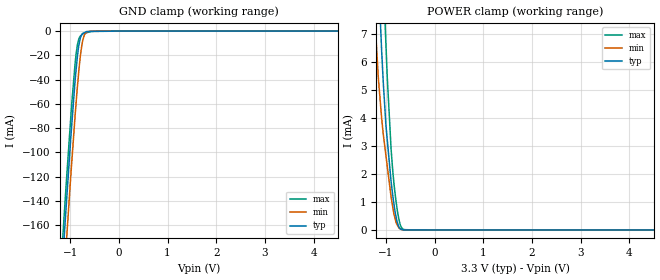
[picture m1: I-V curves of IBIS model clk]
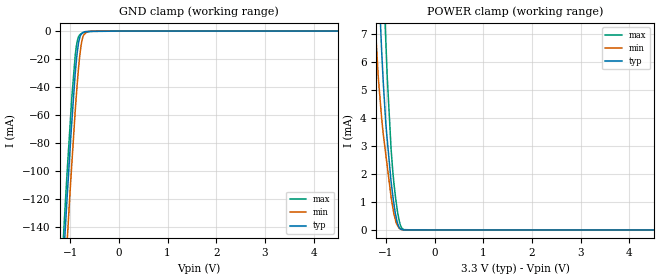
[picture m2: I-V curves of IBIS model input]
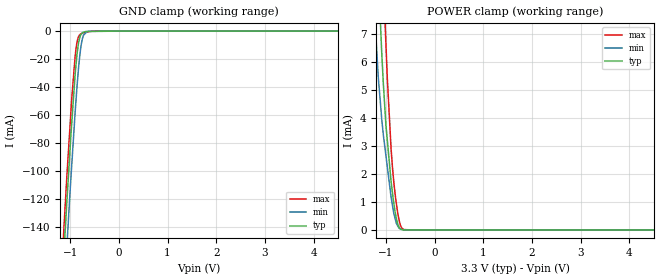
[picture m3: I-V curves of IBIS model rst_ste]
|Texas Instruments Incorporated
| A LOW COST INTEGRATED ANALOG FRONT END FOR WEIGH SCALE AND BODY COMPOSITION
| MEASUREMENT
| Marketing part#   Digital Voltage Range   Package-type   #pins
| AFE4300   2.0V - 3.6V   TQFP   80
[IBIS Ver]   3.2
[File name]   afe4300pn.ibs
[File Rev]   1.0
[Date]   6/8/2012
[Source]
| Texas Instruments Incorporated.
| Analog-eLab Design Center, HPA
| 12500 TI Blvd
| Dallas, TX -75243
| e-mail: elab_scm_ibis@list.ti.com
[Notes]   Revision History:
| Rev 1.0: 6/8/2012
| - Initial version of the model
| - Model generated from simulations in TISPICE
| - Model matched to SPICE simulation
| - C_comp although listed in numerical order of value are
|   obtained from varying PVT conditions. For PVT conditions for
|   each specific value refer the buffer description under
|   respective [Model]. IBIS model user is responsible for using
|   appropriate C_comp to simulate for Signal Integrity.
| - Model names with a trailing _3p3 contains the model for
|   3.3V [3.0V and 3.6V].
[Disclaimer]
| This model is designed as an aid for customers of Texas Instruments.
| TI and its licensors and suppliers make no warranties, either expressed
| or implied, with respect to this  model, including the warranties of
| merchantability or fitness for a particular purpose. The model is
| provided solely on an "as is" basis. The entire risk as to its quality
| and performance is with the customer.
[Copyright]
 (C) Copyright 2011 Texas Instruments Incorporated.All rights reserved.
|   AFE4300PN
[Component]   AFE4300PN
[Manufacturer]   TI
[Package]   |80 TQFP   -  PN package
|   typ   min   max
R_pkg   0.10791   0.08655   0.13328
L_pkg   4.92072nH   4.19191nH   6.00445nH
C_pkg   0.77225pF   0.63735pF   1.07420pF
[Pin]  signal_name   model_name   R_pin   L_pin   C_pin
1   AVSS   gnd   0.06488   4.97502nH  0.79351pF
2   INP1   term   0.12382   5.42900nH  0.85172pF
3   INM1   term   0.12069   5.27719nH  0.83213pF
4   INP2   term   0.11830   5.14232nH  0.81045pF
5   INM2   term   0.11658   5.03610nH  0.79047pF
6   AVSS   gnd   0.11574   4.97329nH  0.71405pF
7   INP_R   term   0.11479   4.85156nH  0.70853pF
8   INM_R   term   0.11470   4.77192nH  0.75908pF
9   AVSS   gnd   0.11737   5.96548nH  1.07056pF
10   INP3   term   0.11594   4.78579nH  0.68513pF
11   INM3   term   0.11660   4.80030nH  0.68657pF
12   INP4   term   0.11918   6.00445nH  1.07420pF
13   INM4   term   0.11809   4.84466nH  0.76427pF
14   AVSS   gnd   0.11963   4.95544nH  0.71226pF
15   AAUX   term   0.12075   5.08150nH  0.70418pF
16   VLDO   term   0.11317   4.96716nH  0.77207pF
17   VREF   term   0.11366   5.04855nH  0.80047pF
18   AVDD   power   0.11453   5.15212nH  0.81475pF
19   DACOUT   term   0.12377   5.43268nH  0.84789pF
20   DAC_FILT_IN   term   0.13328   5.76711nH  0.74859pF
21   AVSS   gnd   0.13115   5.73004nH  0.74408pF
22   IOUT5   term   0.12643   5.49576nH  0.86054pF
23   IOUT4   term   0.12223   5.32047nH  0.84033pF
24   IOUT3   term   0.11875   5.16170nH  0.81605pF
25   IOUT2   term   0.11590   5.03136nH  0.79392pF
26   IOUT1   term   0.11367   4.93832nH  0.71474pF
27   IOUT0   term   0.11178   4.79271nH  0.70623pF
28   RP1   term   0.11064   4.69143nH  0.75471pF
29   RP0   term   0.11208   5.85943nH  1.06436pF
30   RN1   term   0.10991   4.66416nH  0.67662pF
31   RN0   term   0.10965   4.65917nH  0.66509pF
32   AVSS   gnd   0.11258   5.87032nH  1.05278pF
33   VSENSE5   term   0.10888   4.65569nH  0.75096pF
34   VSENSE4   term   0.10764   4.70739nH  0.69961pF
35   VSENSE3   term   0.10712   4.79958nH  0.70339pF
36   VSENSE2   term   0.10696   4.84185nH  0.77759pF
37   VSENSE1   term   0.10745   4.92272nH  0.79503pF
38   VSENSE0   term   0.10865   5.03281nH  0.81479pF
39   VSENSEP_R1   term   0.11067   5.16161nH  0.83129pF
40   VSENSEP_R0   term   0.11360   5.35645nH  0.71822pF
41   VSENSEM_R1   term   0.10765   5.23060nH  0.71458pF
42   VSENSEM_R0   term   0.09674   4.87022nH  0.80715pF
43   NC   nc   0.09741   4.79802nH  0.79221pF
44   NC   nc   0.09371   4.63612nH  0.77888pF
45   AVSS   gnd   0.09092   4.50774nH  0.75677pF
46   AVDD   power   0.08905   4.42347nH  0.67917pF
47   OUTM_I_FILT   term   0.08798   4.29859nH  0.67325pF
48   OUTP_I_FILT   term   0.08732   4.20648nH  0.72239pF
49   OUTM_Q_FILT   term   0.08936   5.38610nH  1.03329pF
50   OUTP_Q_FILT   term   0.08789   4.20454nH  0.64654pF
51   AAUX2   term   0.08803   4.20667nH  0.63735pF
52   NC   nc   0.00742   3.98391nH  0.92611pF
53   _RESET   rst_ste   0.08675   4.19191nH  0.70875pF
54   STE   rst_ste   0.08674   4.26853nH  0.65925pF
55   NC   nc   0.00583   2.99607nH  0.56984pF
56   SDOUT   output   0.08722   4.42874nH  0.74037pF
57   SDIN   input   0.08862   4.52766nH  0.76099pF
58   SCLK   input   0.08655   4.57061nH  0.77680pF
59   RDY   output   0.08826   4.69216nH  0.79488pF
60   AVSS   gnd   0.08879   4.83658nH  0.67875pF
61   NC   nc   0.00646   3.43131nH  0.58837pF
62   NC   nc   0.00634   3.29482nH  0.69454pF
63   NC   nc   0.00622   3.20561nH  0.68015pF
64   NC   nc   0.00608   3.11757nH  0.66177pF
65   NC   nc   0.00595   3.04425nH  0.64463pF
66   NC   nc   0.00583   2.99602nH  0.56986pF
67   NC   nc   0.00536   2.86106nH  0.56090pF
68   NC   nc   0.00532   2.79061nH  0.60735pF
69   NC   nc   0.00733   3.97085nH  0.91820pF
70   NC   nc   0.00533   2.78774nH  0.53745pF
71   NC   nc   0.00536   2.79295nH  0.53912pF
72   NC   nc   0.08978   5.38902nH  1.01684pF
73   NC   nc   0.08745   4.20291nH  0.71651pF
74   NC   nc   0.08899   4.31242nH  0.66607pF
75   NC   nc   0.08705   4.37168nH  0.66100pF
76   NC   nc   0.00591   3.03491nH  0.64624pF
77   AVSS   gnd   0.08838   4.50833nH  0.74945pF
78   NC   nc   0.00613   3.18898nH  0.67809pF
79   CLK   clk   0.09735   4.85821nH  0.80082pF
80   AVDD   power   0.10961   5.24317nH  0.71225pF
[Model] term
Model_type Terminator
C_comp   1.0e-20F  1.0e-20F  1.0e-20F
|   typ   min   max
[Voltage Range]   3.3V   3.0V   3.6V
[POWER Clamp Reference]   3.3V   3.0V   3.6V
[GND Clamp Reference]   0V   0V   0V
|Ambient Temperature   25   70   0
|Junction Temperature
[Temperature Range]   27   70   0
| Models and submodels in the file (5): clk (Input), input (Input), rst_ste (Input), output (3-state), term (Terminator)
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|   clk Model
[Model]   clk
Model_type   Input
Vinl = 0.825
Vinh = 2.475
|   typ   min   max
|   (nom PVT)   (fast PVT)   (slow PVT)
|C_comp from frequency sweep method (F=1MHz)
|Average
|C_comp   1.741e-12   1.543e-12   1.951e-12
|C_comp from LC tank measurement(L=1nH)
|Average
|Resonant Frequency(Hz)   4.160e+09   4.370e+09   3.990e+09
 C_comp   1.465e-12   1.328e-12   1.593e-12
| Where nom  PVT is Nominal Process, 3.3V, 27C
|   Fast PVT is Strong Process,  3.6V, 0C
|   Slow PVT is Weak Process,   3V, 70C
[Voltage Range]   3.3   3   3.6
|Ambient Temperature   25   70   0
|Junction Temperature
[Temperature Range]   27   70   0
[Power Clamp Reference]   3.3   3   3.6
[GND Clamp Reference]   0   0   0
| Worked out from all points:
|   GND clamp passes 1 mA (typ) near -0.70 V on its own axis
|   POWER clamp passes 1 mA (typ) near -0.84 V on its own axis
[GND Clamp]
|   Voltage   I(typ)   I(min)   I(max)
-3.3V     -1.639A    -1.658A    -1.629A
-1.242V   -245.7mA   -276.8mA   -227.9mA
-1.134V   -176.7mA   -208.5mA   -158.7mA
-1.112V   -162.8mA   -194.9mA   -145.1mA
-1.08V    -143.5mA   -175mA     -125.1mA
-972mV    -79.57mA   -110.4mA   -61.99mA
-874.8mV  -30.33mA   -57.42mA   -17.78mA
-821.7mV  -11.6mA    -32.45mA   -6.684mA
-765mV    -3.159mA   -12.81mA   -3.212mA
-711mV    -1.283mA   -3.46mA    -1.91mA
-663.3mV  -394.4uA   -1.035mA   -1.359mA
6.6V      0A         0A         0A
[POWER Clamp]
|   Voltage   I(typ)   I(min)   I(max)
-3.3V     115.8mA    98.78mA    130.3mA
-1.214V   11.39mA    7.085mA    16.78mA
-1.158V   9.11mA     5.413mA    13.92mA
-1.092V   6.453mA    4.029mA    10.6mA
-1.056V   5.225mA    3.394mA    8.928mA
-1.003V   3.746mA    2.657mA    6.649mA
-975.6mV  3.222mA    2.273mA    5.458mA
-896.4mV  1.721mA    1.17mA     2.883mA
-867.6mV  1.31mA     872.4uA    2.216mA
-778.8mV  327.2uA    202uA      824.3uA
-702mV    39.25uA    27.21uA    154.8uA
6.6V      0A         0A         0A
|   input Model
[Model]   input
Model_type   Input
Vinl = 0.825
Vinh = 2.475
|   typ   min   max
|   (nom PVT)   (fast PVT)   (slow PVT)
|C_comp from frequency sweep method (F=4MHz)
|Average
|C_comp   1.194e-12   1.058e-12   1.336e-12
|C_comp from LC tank measurement(L=1nH)
|Average
|Resonant Frequency(Hz)   5.270e+09   5.430e+09   5.150e+09
 C_comp   9.130e-13   8.599e-13   9.560e-13
| Where nom  PVT is Nominal Process, 3.3V, 27C
|   Fast PVT is Strong Process,  3.6V, 0C
|   Slow PVT is Weak Process,   3V, 70C
[Voltage Range]   3.3   3   3.6
|Ambient Temperature   25   70   0
|Junction Temperature
[Temperature Range]   27   70   0
[Power Clamp Reference]   3.3   3   3.6
[GND Clamp Reference]   0   0   0
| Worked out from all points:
|   GND clamp passes 1 mA (typ) near -0.74 V on its own axis
|   POWER clamp passes 1 mA (typ) near -0.84 V on its own axis
[GND Clamp]
|   Voltage   I(typ)   I(min)   I(max)
-3.3V     -1.598A    -1.621A    -1.586A
-1.22V    -216.1mA   -248.6mA   -197.5mA
-1.122V   -154.6mA   -186.2mA   -137mA
-1.102V   -142.5mA   -174.4mA   -124.9mA
-1.066V   -120.7mA   -152.6mA   -102.4mA
-968.4mV  -66mA      -96.14mA   -48.5mA
-896.4mV  -30.3mA    -57.15mA   -17.38mA
-825mV    -7.646mA   -25.28mA   -3.826mA
-777mV    -2.539mA   -10.58mA   -1.914mA
-726mV    -710.4uA   -2.929mA   -1.242mA
-576mV    -276.4uA   -38.12uA   -169.3uA
6.6V      0A         0A         0A
[POWER Clamp]
|   Voltage   I(typ)   I(min)   I(max)
-3.3V     115.8mA    98.78mA    130.3mA
-1.214V   11.39mA    7.085mA    16.78mA
-1.158V   9.11mA     5.413mA    13.92mA
-1.092V   6.453mA    4.029mA    10.6mA
-1.056V   5.225mA    3.394mA    8.928mA
-1.003V   3.746mA    2.657mA    6.649mA
-975.6mV  3.222mA    2.273mA    5.458mA
-896.4mV  1.721mA    1.17mA     2.883mA
-867.6mV  1.31mA     872.4uA    2.216mA
-778.8mV  327.2uA    202uA      824.3uA
-702mV    39.25uA    27.21uA    154.8uA
6.6V      0A         0A         0A
|   rst_ste Model
[Model]   rst_ste
Model_type   Input
Vinl = 0.825
Vinh = 2.475
|   typ   min   max
|   (nom PVT)   (fast PVT)   (slow PVT)
|C_comp from frequency sweep method (F=4MHz)
|Average
|C_comp   1.174e-12   1.046e-12   1.308e-12
|C_comp from LC tank measurement(L=1nH)
|Average
|Resonant Frequency(Hz)   5.270e+09   5.430e+09   5.150e+09
 C_comp   9.130e-13   8.599e-13   9.560e-13
| Where nom  PVT is Nominal Process, 3.3V, 27C
|   Fast PVT is Strong Process,  3.6V, 0C
|   Slow PVT is Weak Process,   3V, 70C
[Voltage Range]   3.3   3   3.6
|Ambient Temperature   25   70   0
|Junction Temperature
[Temperature Range]   27   70   0
[Power Clamp Reference]   3.3   3   3.6
[GND Clamp Reference]   0   0   0
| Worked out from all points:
|   GND clamp passes 1 mA (typ) near -0.74 V on its own axis
|   POWER clamp passes 1 mA (typ) near -0.84 V on its own axis
[GND Clamp]
|   Voltage   I(typ)   I(min)   I(max)
-3.3V     -1.598A    -1.621A    -1.586A
-1.22V    -216.1mA   -248.6mA   -197.5mA
-1.122V   -154.6mA   -186.2mA   -137mA
-1.102V   -142.5mA   -174.4mA   -124.8mA
-1.066V   -120.7mA   -152.6mA   -102.4mA
-968.4mV  -66mA      -96.14mA   -48.5mA
-896.4mV  -30.3mA    -57.15mA   -17.38mA
-825mV    -7.644mA   -25.28mA   -3.822mA
-777mV    -2.537mA   -10.58mA   -1.912mA
-726mV    -709uA     -2.928mA   -1.24mA
-576mV    -275.5uA   -37.7uA    -168.6uA
6.6V      0A         0A         0A
[POWER Clamp]
|   Voltage   I(typ)   I(min)   I(max)
-3.3V     115.9mA    98.8mA     130.4mA
-1.214V   11.4mA     7.089mA    16.78mA
-1.158V   9.114mA    5.416mA    13.93mA
-1.092V   6.457mA    4.032mA    10.6mA
-1.056V   5.228mA    3.396mA    8.932mA
-1.003V   3.749mA    2.66mA     6.652mA
-975.6mV  3.224mA    2.275mA    5.46mA
-896.4mV  1.723mA    1.172mA    2.885mA
-867.6mV  1.312mA    873.9uA    2.217mA
-778.8mV  327.9uA    202.9uA    825uA
-702mV    39.52uA    27.77uA    155.1uA
6.6V      0A         0A         0A
